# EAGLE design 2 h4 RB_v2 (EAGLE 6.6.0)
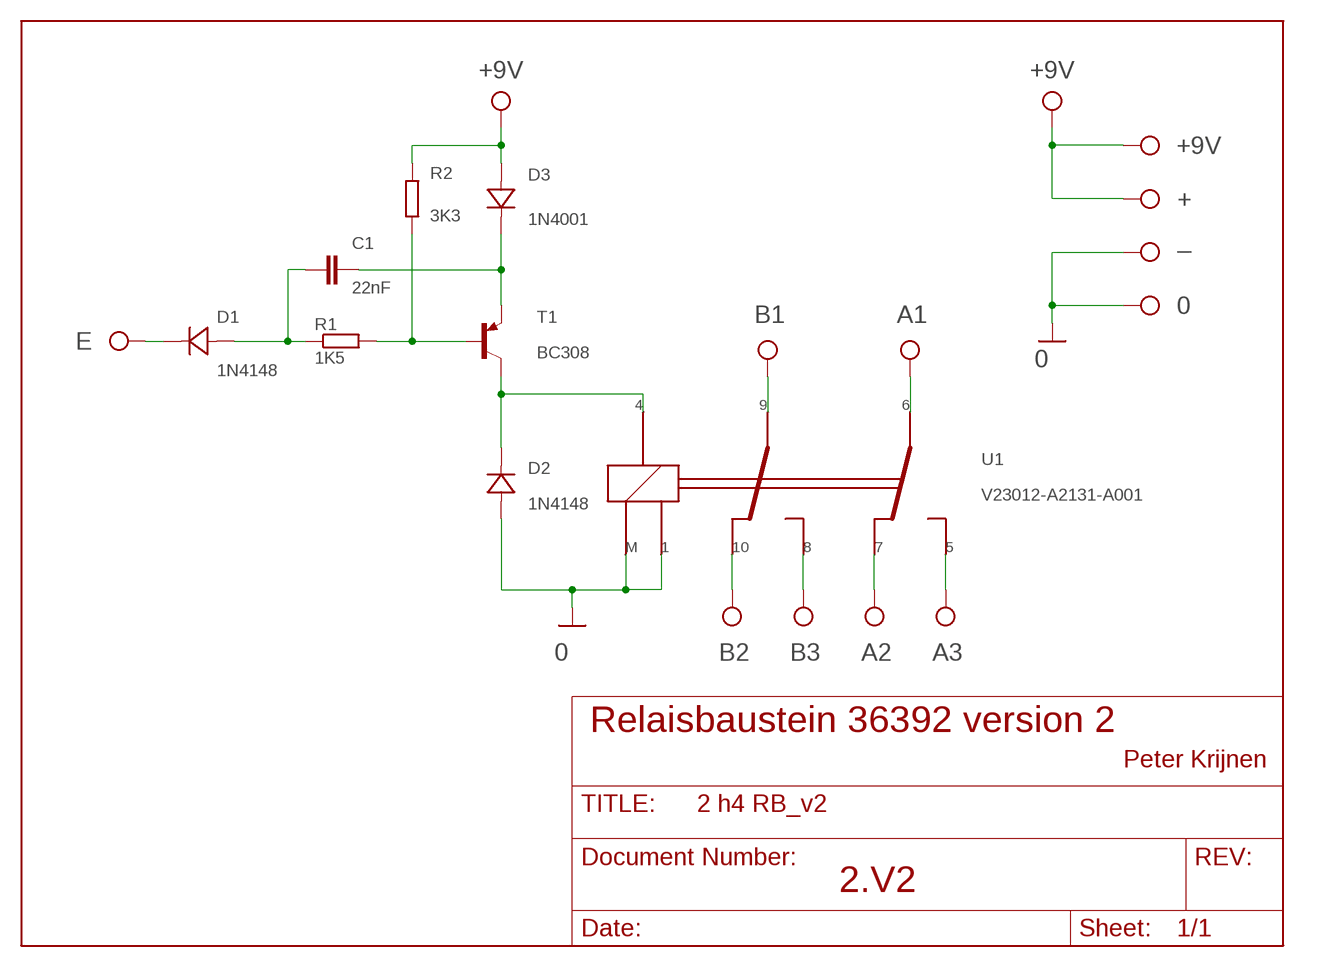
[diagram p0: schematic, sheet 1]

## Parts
0  PIN_2  [PIN_2]
+  SMD5  [SMD2,54-5,08]
+9V  PIN_2  [PIN_2]
_  SMD5  [SMD2,54-5,08]
A1  PIN_2  [PIN_2]
A2  PIN_2  [PIN_2]
A3  PIN_2  [PIN_2]
B1  PIN_2  [PIN_2]
B2  PIN_2  [PIN_2]
B3  PIN_2  [PIN_2]
C1  22nF  C-EU050-025X075  [C050-025X075]
D1  1N4148  DIODE-7.5  [D-7.5]
D2  1N4148  DIODE-7.5  [D-7.5]
D3  1N4001  DIODE-10  [D-10]
E  PIN_2  [PIN_2]
R1  1K5  R-EU_0207/10  [0207/10]
R2  3K3  R-EU_0207/10  [0207/10]
T1  BC308  FT-PNP  [FT-PNP]
U1  V23012-A2131-A001  V23012-A2131  [V23012]

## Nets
E: D1.K(C) E.P$1
GND: 0.P$1 _.1(P) D2.A U1.1 U1.M ; supply symbol labelled 0
N$1: B2.P$1 U1.10
N$2: B3.P$1 U1.8
N$3: A2.P$1 U1.7
N$4: A3.P$1 U1.5
N$5: A1.P$1 U1.6
N$6: B1.P$1 U1.9
N$8: C1.2 D1.A R1.1
N$11: R1.2 R2.1 T1.2(B)
N$14: C1.1 D3.K(C) T1.1(E)
N$15: D2.K(C) T1.3(C) U1.4
VCC: +9V.P$1 +.1(P) D3.A R2.2 ; supply symbol labelled +9V

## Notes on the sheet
- Relaisbaustein 36392 version 2
- Peter Krijnen
- 2.V2

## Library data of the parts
0 +9V A1-A3 B1-B3 E = ft_spec:PIN_2
+ _ = wirepad:SMD5: SMD PAD
C1 = rcl:C-EU: CAPACITOR, European symbol
D1-D3 = diode:DIODE-: DIODE
R1 R2 = rcl:R-EU_: RESISTOR, European symbol
T1 = transistor-pnp:FT-PNP
U1 = FT-SPEC:V23012

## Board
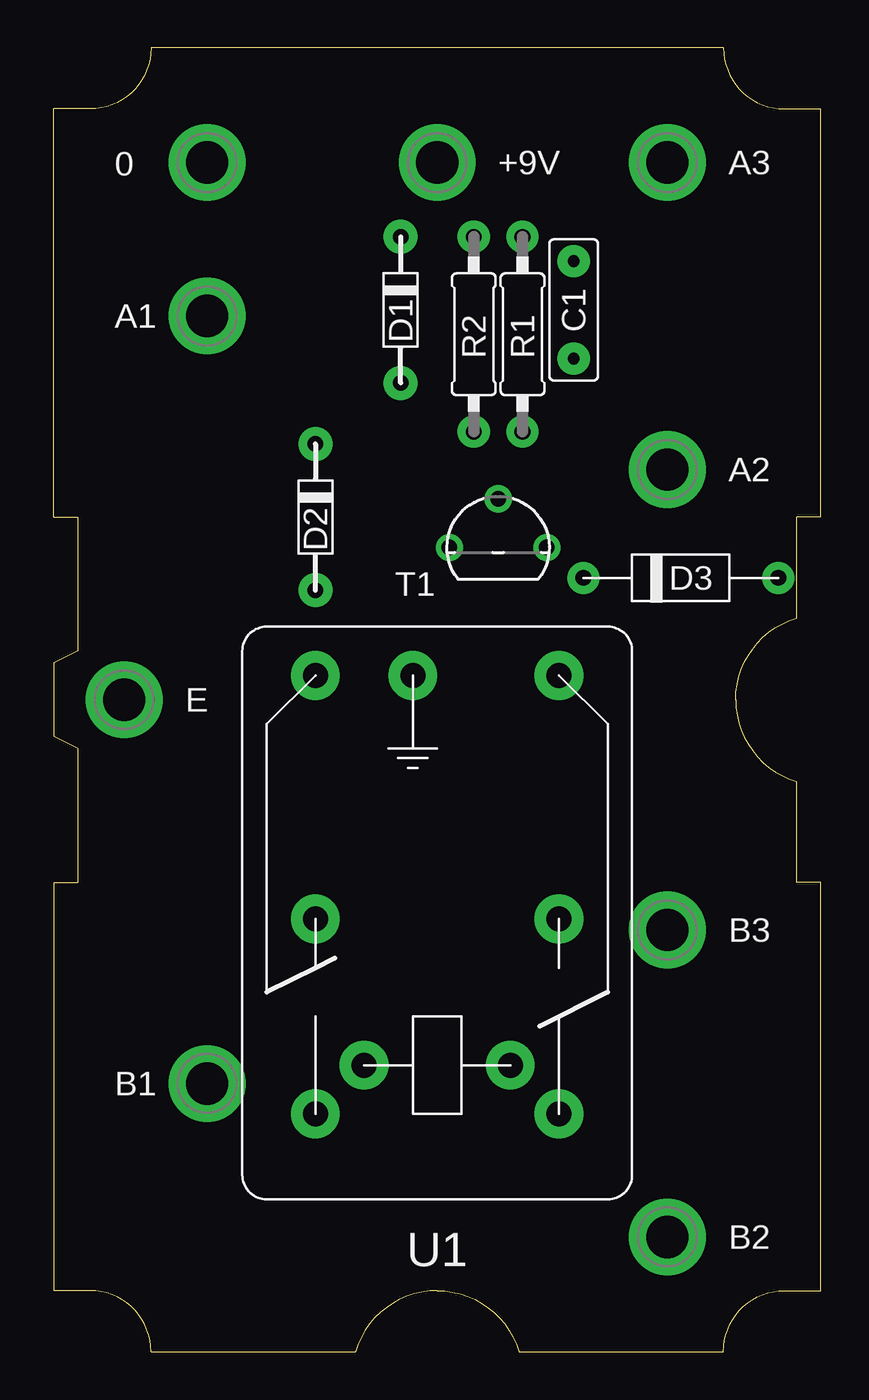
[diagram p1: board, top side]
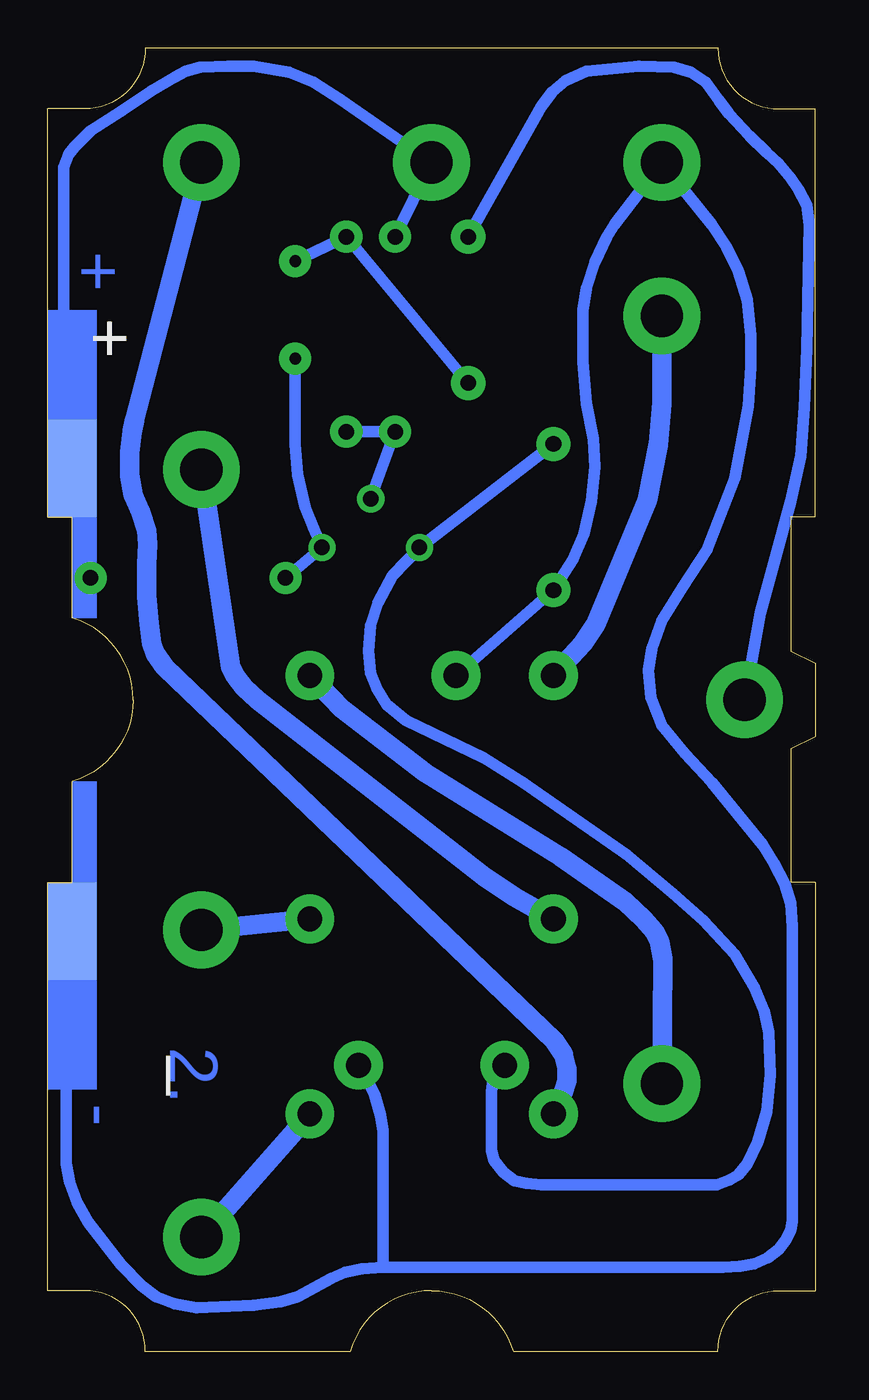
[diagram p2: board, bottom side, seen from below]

Size 40.01 x 67.94 mm. Coordinates in mm from the lower left corner, seen from the top.
Copper layers 16: Bottom 0.035mm
Design rules "default": minimum track width 10mil, minimum drill 24mil, track to track 8mil, track to pad 8mil, pad to pad 8mil, via to via 8mil, smd to smd 8mil, copper to edge 0.25mm, drill to drill 8mil, minimum pad ring 10mil, minimum via ring 8mil, stop-mask expansion 0mil, vias tented up to drill 0mil, thermal gap 10mil

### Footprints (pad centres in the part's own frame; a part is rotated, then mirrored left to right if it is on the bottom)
PIN_2 = drill 2.2 pad 4: P$1 0,0
SMD2,54-5,08 = smd 2.54 x 5.08: 1 0,0
C050-025X075 = drill 0.61 pad 1.676: 1 -2.54,0; 2 2.54,0
D-7.5 = drill 0.813 pad 1.778: A -3.81,0; K 3.81,0
D-10 = drill 0.813 pad 1.676: A -5.08,0; K 5.08,0
0207/10 = drill 0.813 pad 1.676: 1 -5.08,0; 2 5.08,0
FT-PNP = drill 0.813 pad 1.422: 1 2.54,0; 2 0,2.54; 3 -2.54,0
V23012 = drill 1.3 pad 2.54: 1 -7.62,-3.81; 4 -7.62,3.81; 5 -10.16,6.35; 6 12.7,6.35; 7 0,6.35; 8 0,-6.35; 9 12.7,-6.35; 10 -10.16,-6.35; M 12.7,1.27

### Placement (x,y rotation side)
0  8,61.98 0 top
+  38.73,46.04 180 bottom
+9V  20,61.98 0 top
_  38.73,21.91 180 bottom
A1  8,53.98 0 top
A2  32,45.97 0 top
A3  32,61.98 0 top
B1  8,13.97 0 top
B2  32,5.97 0 top
B3  32,21.97 0 top
C1  27.11,54.29 90 top
D1  18.1,54.29 90 top
D2  13.65,43.5 90 top
D3  32.7,40.32 180 top
E  3.68,33.97 0 top
R1  24.45,53.02 270 top
R2  21.91,53.02 90 top
T1  23.18,41.91 0 top
U1  20,22.54 90 top
U$1  [PRINTFORM_4575]  40.01,-0.95 90 top
U$5  [DIM_4070]  40.01,0 90 top

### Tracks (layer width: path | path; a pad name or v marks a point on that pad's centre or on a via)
E
  Bottom 0.61: D1.K 14.29,64.9 13.72,65.66 13.02,66.23 11.94,66.74 9.21,66.99 7.37,66.93 6.48,66.67 5.71,66.17 5.02,65.22 4.51,64.52 3.43,63.37 2.54,62.48 1.91,61.91 1.27,61.15 0.89,60.58 0.45,59.75 0.32,58.74 0.45,52.26 0.57,49.21 0.76,46.67 1.27,44.32 2.16,41.08 2.86,38.48 3.24,36.45 E.P$1
GND
  Bottom 0.61: U1.M D2.A 12.64,41.27 12.06,42.61 11.68,44.32 11.49,46.1 11.56,47.56 11.94,49.4 12.13,51.56 12.13,54.29 11.94,55.44 11.49,56.77 10.86,58.1 10.48,58.74 0.P$1 5.4,58.74 4.64,57.59 4,56.33 3.56,54.8 3.37,52.96 3.37,51.31 3.49,49.28 4.19,45.53 5.65,41.78 6.92,39.81 8,38.1 8.51,36.64 8.7,35.5 8.57,34.1 8,32.64 6.79,31.18 5.4,29.65 2.73,26.42 2.16,25.46 1.59,24.38 1.27,23.37 1.21,22.16 1.21,6.79 1.27,6.35 1.52,5.84 1.91,5.33 2.48,4.89 3.17,4.57 3.94,4.45 4.83,4.38 22.54,4.38 | 22.54,4.38 23.62,4.32 24.51,4.13 25.21,3.81 26.99,2.86 27.88,2.6 29.27,2.41 32.26,2.29 33.4,2.48 34.35,2.86 35.12,3.43 36.2,4.51 37.91,6.73 38.48,7.75 38.86,8.83 39.05,9.78 39.05,21.59 arc90 _.1 | 22.54,4.38 22.54,11.49 22.67,12.32 22.99,13.4 23.43,14.29 U1.1
N$1
  Bottom 1.016: U1.10 B2.P$1
N$2
  Bottom 1.016: B3.P$1 U1.8
N$3
  Bottom 1.016: U1.7 15.68,23.69 17.27,24.77 29.08,33.97 29.78,34.61 30.23,35.18 30.48,35.69 A2.P$1
N$4
  Bottom 1.016: U1.5 13.14,13.53 12.95,14.1 12.95,14.73 13.14,15.49 13.59,16.19 33.91,35.69 34.42,36.39 34.61,36.89 34.73,37.91 34.86,39.37 34.86,41.02 34.8,42.1 34.86,42.8 35.18,43.75 35.56,44.64 35.75,45.66 35.75,46.86 35.62,47.94 35.5,48.58 A3.P$1
N$5
  Bottom 1.016: U1.6 12.13,36.89 11.43,37.91 8.76,44.39 8.19,47.31 8,49.4 A1.P$1
N$6
  Bottom 1.016: U1.9 24.7,33.53 20.32,30.16 13.27,25.78 9.91,23.43 8.95,22.54 8.38,21.91 8.13,21.4 7.94,20.45 B1.P$1
N$8
  Bottom 0.61: D1.A R1.1 C1.2
N$11
  Bottom 0.61: R1.2 R2.1 T1.2
N$14
  Bottom 0.61: C1.1 27.11,47.31 26.99,45.72 26.61,44.01 26.16,42.93 T1.1 D3.K
N$15
  Bottom 0.61: U1.4 16.64,14.41 16.83,13.97 16.89,13.53 16.89,10.48 16.76,9.97 16.26,9.34 15.68,8.89 15.05,8.76 14.29,8.7 5.14,8.7 4.45,8.95 4,9.21 3.56,9.78 2.98,10.92 2.54,12.51 2.35,14.41 2.41,16.64 2.67,17.72 3.17,18.99 4.19,20.7 5.84,22.48 7.43,23.88 9.84,25.91 15.24,29.65 17.27,30.92 21.34,32.89 22.35,33.72 22.86,34.54 23.18,35.37 23.3,36.51 23.18,37.85 22.8,39.05 22.04,40.45 T1.3 D2.K
VCC
  Bottom 0.61: D3.A 37.78,45.09 +.1 39.18,46.48 39.18,61.72 38.92,62.42 38.61,62.8 37.78,63.63 36.2,64.64 34.61,65.72 33.4,66.42 32.83,66.74 32.07,66.93 30.61,66.99 29.27,66.99 27.43,66.67 26.16,66.17 24.77,65.28 +9V.P$1 R2.2
(copper drawn outside any net)
  shapes: Bottom area x4

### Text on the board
Bottom: + | 2. | -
